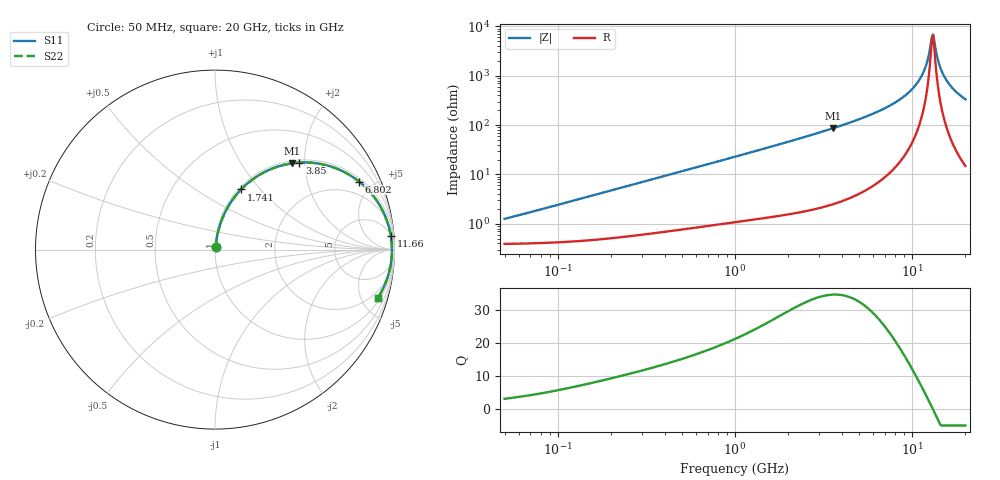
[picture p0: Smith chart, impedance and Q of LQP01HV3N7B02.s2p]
!Murata Part Number: LQP01HV3N7B02
!These Parameters are Measured in Series Mode Connection
!  o--[Z]--o
!Port1  Port2
!  o-------o
!Freq. Start=50[MHz] Stop=20[GHz], 401[Steps]
# Hz S RI R 50
!Freq.(Hz) S11(Real) S11(Imag) S21(Real) S21(Imag) S12(Real) S12(Imag) S22(Real) S22(Imag)
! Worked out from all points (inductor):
!   401 points, 50 MHz to 20 GHz, reference 50 ohm
!   read as one part in series: L = 3.82 nH near 51.52 MHz
!   highest Q = 34.6 at 3.572 GHz (marker M1), where L = 3.84 nH
!   self-resonance near 12.95 GHz
!   S11 on the Smith chart (normalised r, x): 50 MHz: 1.01, +0.02; 1.741 GHz: 1.03, +0.80; 3.85 GHz: 1.05, +1.88; 6.802 GHz: 1.16, +4.15; 11.66 GHz: 6, +24; 20 GHz: 1.30, -6.66
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5e7  0.00405 0.0119  0.996 -0.0119  0.996 -0.0119  0.00405 0.0119
1.364002e8  0.00554 0.0322  0.9945 -0.0322  0.9945 -0.0322  0.00554 0.0322
3.721004e8  0.0139 0.0849  0.9861 -0.0849  0.9861 -0.0849  0.0139 0.0849
1e9  0.0587 0.2126  0.9413 -0.2126  0.9413 -0.2126  0.0587 0.2126
1.740566e9  0.1458 0.3354  0.8542 -0.3354  0.8542 -0.3354  0.1458 0.3354
2.728004e9  0.295 0.4412  0.705 -0.4412  0.705 -0.4412  0.295 0.4412
3.572216e9  0.4284 0.4806  0.5716 -0.4806  0.5716 -0.4806  0.4284 0.4806
3.850025e9  0.4705 0.4849  0.5295 -0.4849  0.5295 -0.4849  0.4705 0.4849
5.117541e9  0.6406 0.4645  0.3594 -0.4645  0.3594 -0.4645  0.6406 0.4645
6.802353e9  0.8026 0.3791  0.1974 -0.3791  0.1974 -0.3791  0.8026 0.3791
7.442007e9  0.8467 0.3393  0.1533 -0.3393  0.1533 -0.3393  0.8467 0.3393
9.892087e9  0.9499 0.1819  0.0501 -0.1819  0.0501 -0.1819  0.9499 0.1819
1.082228e10  0.969 0.1252  0.031 -0.1252  0.031 -0.1252  0.969 0.1252
1.166392e10  0.9796 0.0764  0.0204 -0.0764  0.0204 -0.0764  0.9796 0.0764
1.220001e10  0.9835 0.0468  0.0165 -0.0468  0.0165 -0.0468  0.9835 0.0468
1.276073e10  0.9856 0.0169  0.0144 -0.0169  0.0144 -0.0169  0.9856 0.0169
1.314879e10  0.9859 -0.00308  0.0141 0.00308  0.0141 0.00308  0.9859 -0.00308
1.334722e10  0.9858 -0.0131  0.0142 0.0131  0.0142 0.0131  0.9858 -0.0131
1.438523e10  0.9822 -0.0629  0.0178 0.0629  0.0178 0.0629  0.9822 -0.0629
1.527346e10  0.9756 -0.1023  0.0244 0.1023  0.0244 0.1023  0.9756 -0.1023
1.721783e10  0.953 -0.179  0.047 0.179  0.047 0.179  0.953 -0.179
2e10  0.9075 -0.2683  0.0925 0.2683  0.0925 0.2683  0.9075 -0.2683
